| IBIS file stm32u375_385_wlcsp68-q_smps.ibs
[IBIS ver] 4.2
[File name] stm32u375_385_wlcsp68-q_smps.ibs
[File Rev] 1.2
[Date] 23-06-2025
[Source] Data Created at STMicroelectronics
[Notes]  File originated from ELDO simulations.
[Disclaimer]  This information is for modeling purpose only and is
   not guaranted. The information is subject to change without
   notice.
[Copyright] Copyright 2025 STMicroelectronics Inc.
|   Component stm32u375_385_wlcsp68-q_smps
[Component] stm32u375_385_wlcsp68-q_smps
[Manufacturer] STMicroelectronics
[Package]
| variable   typ   min   max
R_pkg  0  NA  NA
L_pkg  0  NA  NA
C_pkg  0  NA  NA
[Pin]   signal_name   model_name
A1  VDD  power
A3  PC12  io8_ft_100m_hslv
A5  PB3  io8_ft_100m_hslv
A7  PH3-BOOT0  io8_ft_100m_hslv
A9  VDD  power
B2  VDDUSB  power
B4  PC11  io8_ft_100m_hslv
B6  PB4  io8_ft_100m_hslv
B8  PB8  io8_ft_100m_hslv
C1  PA12  io8usb_ft_phy
C3  PA14  io8_ft_100m
C5  PD2  io8_ft_100m_hslv
C7  PB7  io8_ft_100m_hslv
C9  PB9  io8_ft_100m_hslv
D2  VSS  gnd
D4  PA15  io8_ft_100m
D6  PB5  io8_ft_100m_hslv
D8  VSS  gnd
E1  PA11  io8usb_ft_phy
E3  PA13  io8_ft_100m
E5  PC10  io8_ft_100m_hslv
E7  PC13  io8_ft_100m_v33
E9  PC14-OSC32_IN  io_ft_tamp
F2  PC9  io8_ft_100m_hslv
F4  PA10  io8_ft_100m
F6  PB6  io8_ft_100m_hslv
F8  PC15-OSC32_OUT  io_ft_tamp
G1  PC8  io8_ft_100m_hslv
G3  PC7  io8_ft_100m_hslv
G5  PA9  io8_ft_100m
G7  PC0  io8_ft_100m_hslv
G9  PH0-OSC_IN  io8_ft_100m
H2  PC6  io8_ft_100m_hslv
H4  PA8  io8_ft_100m_hslv
H6  PC1  io8_ft_100m_hslv
H8  PH1-OSC_OUT  io8_ft_100m
J1  PD13  io8_ft_100m_hslv
J3  PD12  io8_ft_100m_hslv
J5  PA6  io8_ft_100m_hslv
J7  PA0  io8_ft_100m
J9  NRST  ioreset_v33
K2  PB15  io8_ft_100m
K4  PB10  io8_ft_100m_hslv
K6  PA2  io8_ft_100m_hslv
K8  PC2  io8_ft_100m_hslv
L1  PB14  io8_ft_100m_hslv
L3  PB13  io8_ft_100m_hslv
L5  PB1  io8_ft_100m_hslv
L7  PA1  io8_ft_100m_hslv
L9  PC3  io8_ft_100m_hslv
M2  PB12  io8_ft_100m_hslv
M4  PB11  io8_ft_100m_hslv
M6  PA5  io8_ft_100m
M8  VSSA  nc
N1  VSS  gnd
N3  VSSSMPS  nc
N5  PB0  io8_ft_100m_hslv
N7  PA3  io8_ft_100m_hslv
N9  VDDA  nc
P2  VDD11  nc
P4  VLXSMPS  nc
P6  PA4  io8_ft_100m_hslv
P8  VSS  gnd
R1  VDD  power
R3  VDDSMPS  nc
R5  PB2  io8_ft_100m_hslv
R7  PA7  io8_ft_100m_hslv
R9  VDD  power
[Package Model]   454-wlcsp68-portg_off-250428
[Pin Mapping]   pulldown_ref   pullup_ref   | Comment
A1  nc  vddio
A3  gndio  vddio
A5  gndio  vddio
A7  gndio  vddio
A9  nc  vddio
B2  nc  vddusb
B4  gndio  vddio
B6  gndio  vddio
B8  gndio  vddio
C1  gndio  vddusb  | Depending on IO usage
| C1  gndio  vddio  | Depending on IO usage
C3  gndio  vddio
C5  gndio  vddio
C7  gndio  vddio
C9  gndio  vddio
D2  gndio  nc
D4  gndio  vddio
D6  gndio  vddio
D8  gndio  nc
E1  gndio  vddusb  | Depending on IO usage
| E1  gndio  vddio  | Depending on IO usage
E3  gndio  vddio
E5  gndio  vddio
E7  gndio  vddio
E9  gndio  vddio
F2  gndio  vddio
F4  gndio  vddio
F6  gndio  vddio
F8  gndio  vddio
G1  gndio  vddio
G3  gndio  vddio
G5  gndio  vddio
G7  gndio  vddio
G9  gndio  vddio
H2  gndio  vddio
H4  gndio  vddio
H6  gndio  vddio
H8  gndio  vddio
J1  gndio  vddio
J3  gndio  vddio
J5  gndio  vddio
J7  gndio  vddio
J9  gndio  vddio
K2  gndio  vddio
K4  gndio  vddio
K6  gndio  vddio
K8  gndio  vddio
L1  gndio  vddio
L3  gndio  vddio
L5  gndio  vddio
L7  gndio  vddio
L9  gndio  vddio
M2  gndio  vddio
M4  gndio  vddio
M6  gndio  vddio
M8  nc  nc
N1  gndio  nc
N3  nc  nc
N5  gndio  vddio
N7  gndio  vddio
N9  nc  nc
P2  nc  nc
P4  nc  nc
P6  gndio  vddio
P8  gndio  nc
R1  nc  vddio
R3  nc  nc
R5  gndio  vddio
R7  gndio  vddio
R9  nc  vddio
|[Diff Pin]  inv_pin  vdiff  tdelay_typ  tdelay_min  tdelay_max
|C1  E1  NA  NA  NA  NA
[Model Selector] io8_ft_100m
io8_ft_100m_ls_1v2  "GPIO 100MHz - 5V tolerant - low speed - 1.2V range"
io8_ft_100m_ls_1v8  "GPIO 100MHz - 5V tolerant - low speed - 1.8V range"
io8_ft_100m_ls_3v3  "GPIO 100MHz - 5V tolerant - low speed - 3.3V range"
io8_ft_100m_ms_1v2  "GPIO 100MHz - 5V tolerant - med speed - 1.2V range"
io8_ft_100m_ms_1v8  "GPIO 100MHz - 5V tolerant - med speed - 1.8V range"
io8_ft_100m_ms_3v3  "GPIO 100MHz - 5V tolerant - med speed - 3.3V range"
io8_ft_100m_fs_1v2  "GPIO 100MHz - 5V tolerant - fast speed - 1.2V range"
io8_ft_100m_fs_1v8  "GPIO 100MHz - 5V tolerant - fast speed - 1.8V range"
io8_ft_100m_fs_3v3  "GPIO 100MHz - 5V tolerant - fast speed - 3.3V range"
io8_ft_100m_hs_1v2  "GPIO 100MHz - 5V tolerant - high speed - 1.2V range"
io8_ft_100m_hs_1v8  "GPIO 100MHz - 5V tolerant - high speed - 1.8V range"
io8_ft_100m_hs_3v3  "GPIO 100MHz - 5V tolerant - high speed - 3.3V range"
[Model Selector] io8_ft_100m_hslv
io8_ft_100m_ls_1v2  "GPIO 100MHz - 5V tolerant - low speed - 1.2V range"
io8_ft_100m_ls_1v8  "GPIO 100MHz - 5V tolerant - low speed - 1.8V range"
io8_ft_100m_ls_3v3  "GPIO 100MHz - 5V tolerant - low speed - 3.3V range"
io8_ft_100m_ms_1v2  "GPIO 100MHz - 5V tolerant - med speed - 1.2V range"
io8_ft_100m_ms_1v8  "GPIO 100MHz - 5V tolerant - med speed - 1.8V range"
io8_ft_100m_ms_3v3  "GPIO 100MHz - 5V tolerant - med speed - 3.3V range"
io8_ft_100m_fs_1v2  "GPIO 100MHz - 5V tolerant - fast speed - 1.2V range"
io8_ft_100m_fs_1v8  "GPIO 100MHz - 5V tolerant - fast speed - 1.8V range"
io8_ft_100m_fs_3v3  "GPIO 100MHz - 5V tolerant - fast speed - 3.3V range"
io8_ft_100m_hs_1v2  "GPIO 100MHz - 5V tolerant - high speed - 1.2V range"
io8_ft_100m_hs_1v8  "GPIO 100MHz - 5V tolerant - high speed - 1.8V range"
io8_ft_100m_hs_3v3  "GPIO 100MHz - 5V tolerant - high speed - 3.3V range"
io8_ft_100m_hslv_ls_1v2  "GPIO 100MHz low voltage optimization - 5V tolerant - low speed - 1.2V range"
io8_ft_100m_hslv_ls_1v8  "GPIO 100MHz low voltage optimization - 5V tolerant - low speed - 1.8V range"
io8_ft_100m_hslv_ls_2v5  "GPIO 100MHz low voltage optimization - 5V tolerant - low speed - 3.3V range"
io8_ft_100m_hslv_ms_1v2  "GPIO 100MHz low voltage optimization - 5V tolerant - med speed - 1.2V range"
io8_ft_100m_hslv_ms_1v8  "GPIO 100MHz low voltage optimization - 5V tolerant - med speed - 1.8V range"
io8_ft_100m_hslv_ms_2v5  "GPIO 100MHz low voltage optimization - 5V tolerant - med speed - 3.3V range"
io8_ft_100m_hslv_fs_1v2  "GPIO 100MHz low voltage optimization - 5V tolerant - fast speed - 1.2V range"
io8_ft_100m_hslv_fs_1v8  "GPIO 100MHz low voltage optimization - 5V tolerant - fast speed - 1.8V range"
io8_ft_100m_hslv_fs_2v5  "GPIO 100MHz low voltage optimization - 5V tolerant - fast speed - 3.3V range"
io8_ft_100m_hslv_hs_1v2  "GPIO 100MHz low voltage optimization - 5V tolerant - high speed - 1.2V range"
io8_ft_100m_hslv_hs_1v8  "GPIO 100MHz low voltage optimization - 5V tolerant - high speed - 1.8V range"
io8_ft_100m_hslv_hs_2v5  "GPIO 100MHz low voltage optimization - 5V tolerant - high speed - 3.3V range"
[Model Selector] io8_ft_100m_v33
io8_ft_100m_v33_ls_1v2  "GPIO_V33 100MHz - 5V tolerant - low speed - 1.2V range"
io8_ft_100m_v33_ls_1v8  "GPIO_V33 100MHz - 5V tolerant - low speed - 1.8V range"
io8_ft_100m_v33_ls_3v3  "GPIO_V33 100MHz - 5V tolerant - low speed - 3.3V range"
io8_ft_100m_v33_ms_1v2  "GPIO_V33 100MHz - 5V tolerant - med speed - 1.2V range"
io8_ft_100m_v33_ms_1v8  "GPIO_V33 100MHz - 5V tolerant - med speed - 1.8V range"
io8_ft_100m_v33_ms_3v3  "GPIO_V33 100MHz - 5V tolerant - med speed - 3.3V range"
io8_ft_100m_v33_fs_1v2  "GPIO_V33 100MHz - 5V tolerant - fast speed - 1.2V range"
io8_ft_100m_v33_fs_1v8  "GPIO_V33 100MHz - 5V tolerant - fast speed - 1.8V range"
io8_ft_100m_v33_fs_3v3  "GPIO_V33 100MHz - 5V tolerant - fast speed - 3.3V range"
io8_ft_100m_v33_hs_1v2  "GPIO_V33 100MHz - 5V tolerant - high speed - 1.2V range"
io8_ft_100m_v33_hs_1v8  "GPIO_V33 100MHz - 5V tolerant - high speed - 1.8V range"
io8_ft_100m_v33_hs_3v3  "GPIO_V33 100MHz - 5V tolerant - high speed - 3.3V range"
[Model Selector] io8usb_ft_phy
io8_ft_100m_ls_1v2  "GPIO 100MHz - 5V tolerant - low speed - 1.2V range"
io8_ft_100m_ls_1v8  "GPIO 100MHz - 5V tolerant - low speed - 1.8V range"
io8_ft_100m_ls_3v3  "GPIO 100MHz - 5V tolerant - low speed - 3.3V range"
io8_ft_100m_ms_1v2  "GPIO 100MHz - 5V tolerant - med speed - 1.2V range"
io8_ft_100m_ms_1v8  "GPIO 100MHz - 5V tolerant - med speed - 1.8V range"
io8_ft_100m_ms_3v3  "GPIO 100MHz - 5V tolerant - med speed - 3.3V range"
io8_ft_100m_fs_1v2  "GPIO 100MHz - 5V tolerant - fast speed - 1.2V range"
io8_ft_100m_fs_1v8  "GPIO 100MHz - 5V tolerant - fast speed - 1.8V range"
io8_ft_100m_fs_3v3  "GPIO 100MHz - 5V tolerant - fast speed - 3.3V range"
io8_ft_100m_hs_1v2  "GPIO 100MHz - 5V tolerant - high speed - 1.2V range"
io8_ft_100m_hs_1v8  "GPIO 100MHz - 5V tolerant - high speed - 1.8V range"
io8_ft_100m_hs_3v3  "GPIO 100MHz - 5V tolerant - high speed - 3.3V range"
io8usb_ft_phy_hs_3v3   "USB full speed"
io8usb_ft_phy_ls_3v3   "USB low speed"
[Model Selector] io_ft_tamp
io_ft_tamp_ls_1v2 "io8_ft tamp low speed @ 1.2V"
io_ft_tamp_ls_1v8 "io8_ft tamp low speed @ 1.8V"
io_ft_tamp_ls_3v3 "io8_ft tamp low speed @ 3.3V"
io_ft_tamp_ms_1v2 "io8_ft tamp med speed @ 1.2V"
io_ft_tamp_ms_1v8 "io8_ft tamp med speed @ 1.8V"
io_ft_tamp_ms_3v3 "io8_ft tamp med speed @ 3.3V"
io_ft_tamp_fs_1v2 "io8_ft tamp fast speed @ 1.2V"
io_ft_tamp_fs_1v8 "io8_ft tamp fast speed @ 1.8V"
io_ft_tamp_fs_3v3 "io8_ft tamp fast speed @ 3.3V"
io_ft_tamp_hs_1v2 "io8_ft tamp high speed @ 1.2V"
io_ft_tamp_hs_1v8 "io8_ft tamp high speed @ 1.8V"
io_ft_tamp_hs_3v3 "io8_ft tamp high speed @ 3.3V"
[Model Selector] ioreset_v33
ioreset_v33_1v2 "Reset PAD. 5V tolerant. 1.2V range"
ioreset_v33_1v8 "Reset PAD. 5V tolerant. 1.8V range"
ioreset_v33_3v3 "Reset PAD. 5V tolerant. 3.3V range"
[Define Package Model]  454-wlcsp68-portg_off-250428
[Manufacturer]  Unknown
[OEM]  Unknown
[Description]  None
[Number Of Pins]  65
[Pin Numbers]
| Pin Num   Terminal Name
J9 | NRST
J7 | PA0
L7 | PA1
K6 | PA2
N7 | PA3
P6 | PA4
M6 | PA5
J5 | PA6
R7 | PA7
H4 | PA8
G5 | PA9
F4 | PA10
E1 | PA11
C1 | PA12
E3 | PA13
C3 | PA14
D4 | PA15
N5 | PB0
L5 | PB1
R5 | PB2
A5 | PB3
B6 | PB4
D6 | PB5
F6 | PB6
C7 | PB7
B8 | PB8
C9 | PB9
K4 | PB10
M4 | PB11
M2 | PB12
L3 | PB13
L1 | PB14
K2 | PB15
G7 | PC0
H6 | PC1
K8 | PC2
L9 | PC3
H2 | PC6
G3 | PC7
G1 | PC8
F2 | PC9
E5 | PC10
B4 | PC11
A3 | PC12
E7 | PC13
E9 | PC14-OSC32_IN
F8 | PC15-OSC32_OUT
C5 | PD2
J3 | PD12
J1 | PD13
G9 | PH0-OSC_IN
H8 | PH1-OSC_OUT
A7 | PH3-BOOT0
P2 | VDD11
A1 | VDD
A9 | VDD
R1 | VDD
R9 | VDD
N9 | VDDA
R3 | VDDSMPS
B2 | VDDUSB
P4 | VLXSMPS
D2 | VSS
M8 | VSSA
N3 | VSSSMPS
|[Merged Pins]  D2
|D8  |  VSS
|N1  |  VSS
|P8  |  VSS
[Model Data]
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[End Model Data]
[End Package Model]
|End [Component]
| Models and submodels in the file (53): io8_ft_100m_fs_1v2 (I/O), io8_ft_100m_fs_1v8 (I/O), io8_ft_100m_fs_3v3 (I/O), io8_ft_100m_hs_1v2 (I/O), io8_ft_100m_hs_1v8 (I/O), io8_ft_100m_hs_3v3 (I/O), io8_ft_100m_hslv_fs_1v2 (I/O), io8_ft_100m_hslv_fs_1v8 (I/O), io8_ft_100m_hslv_fs_2v5 (I/O), io8_ft_100m_hslv_hs_1v2 (I/O), io8_ft_100m_hslv_hs_1v8 (I/O), io8_ft_100m_hslv_hs_2v5 (I/O), io8_ft_100m_hslv_ls_1v2 (I/O), io8_ft_100m_hslv_ls_1v8 (I/O), io8_ft_100m_hslv_ls_2v5 (I/O), io8_ft_100m_hslv_ms_1v2 (I/O), io8_ft_100m_hslv_ms_1v8 (I/O), io8_ft_100m_hslv_ms_2v5 (I/O), io8_ft_100m_ls_1v2 (I/O), io8_ft_100m_ls_1v8 (I/O), io8_ft_100m_ls_3v3 (I/O), io8_ft_100m_ms_1v2 (I/O), io8_ft_100m_ms_1v8 (I/O), io8_ft_100m_ms_3v3 (I/O), io8_ft_100m_v33_fs_1v2 (I/O), io8_ft_100m_v33_fs_1v8 (I/O), io8_ft_100m_v33_fs_3v3 (I/O), io8_ft_100m_v33_hs_1v2 (I/O), io8_ft_100m_v33_hs_1v8 (I/O), io8_ft_100m_v33_hs_3v3 (I/O), io8_ft_100m_v33_ls_1v2 (I/O), io8_ft_100m_v33_ls_1v8 (I/O), io8_ft_100m_v33_ls_3v3 (I/O), io8_ft_100m_v33_ms_1v2 (I/O), io8_ft_100m_v33_ms_1v8 (I/O), io8_ft_100m_v33_ms_3v3 (I/O), io8usb_ft_phy_hs_3v3 (I/O), io8usb_ft_phy_ls_3v3 (I/O), io_ft_tamp_fs_1v2 (I/O), io_ft_tamp_fs_1v8 (I/O), io_ft_tamp_fs_3v3 (I/O), io_ft_tamp_hs_1v2 (I/O), io_ft_tamp_hs_1v8 (I/O), io_ft_tamp_hs_3v3 (I/O), io_ft_tamp_ls_1v2 (I/O), io_ft_tamp_ls_1v8 (I/O), io_ft_tamp_ls_3v3 (I/O), io_ft_tamp_ms_1v2 (I/O), io_ft_tamp_ms_1v8 (I/O), io_ft_tamp_ms_3v3 (I/O), ioreset_v33_1v2 (I/O_open_drain), ioreset_v33_1v8 (I/O_open_drain), ioreset_v33_3v3 (I/O_open_drain)
